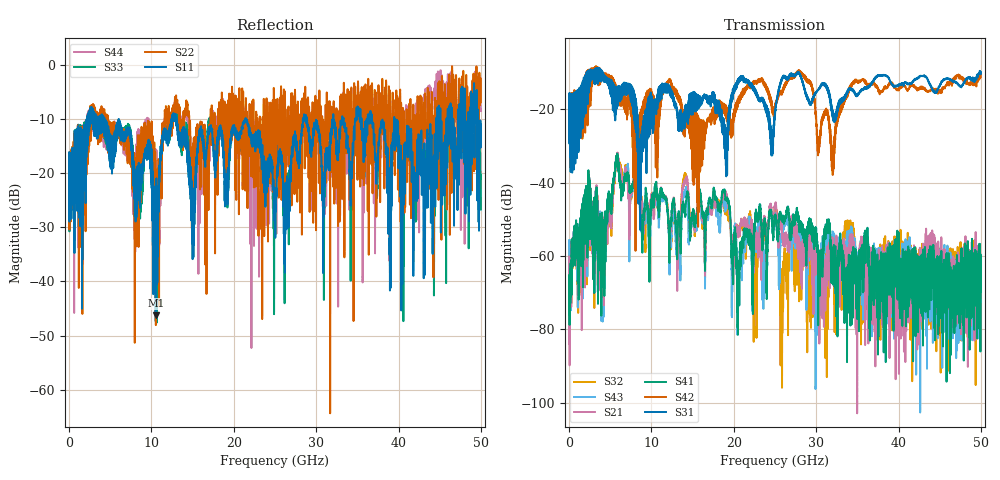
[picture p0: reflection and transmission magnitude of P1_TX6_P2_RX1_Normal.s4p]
!Keysight Technologies,N5225B,MY57041031,A.13.20.10
!Date: Friday, May 31, 2019 11:28:39
!Correction: S11(Full 4 Port(1,2,3,4))
!S12(Full 4 Port(1,2,3,4))
!S13(Full 4 Port(1,2,3,4))
!S14(Full 4 Port(1,2,3,4))
!S21(Full 4 Port(1,2,3,4))
!S22(Full 4 Port(1,2,3,4))
!S23(Full 4 Port(1,2,3,4))
!S24(Full 4 Port(1,2,3,4))
!S31(Full 4 Port(1,2,3,4))
!S32(Full 4 Port(1,2,3,4))
!S33(Full 4 Port(1,2,3,4))
!S34(Full 4 Port(1,2,3,4))
!S41(Full 4 Port(1,2,3,4))
!S42(Full 4 Port(1,2,3,4))
!S43(Full 4 Port(1,2,3,4))
!S44(Full 4 Port(1,2,3,4))
!S4P File: Measurements: <S11,S12,S13,S14>,
!<S21,S22,S23,S24>,
!<S31,S32,S33,S34>,
!<S41,S42,S43,S44>:
# Hz S  dB  R 50.0
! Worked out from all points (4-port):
!   5000 points, 10 MHz to 50 GHz, reference 50 ohm
!   strongest paths, dB at 10 MHz, 12.51 GHz, 25.01 GHz, 37.51 GHz, 50 GHz:
!     S31: -19.4, -15.4, -21.6, -10.8, -9.9
!     S42: -19.4, -14.2, -20.1, -14.4, -10.4
!     S41: -66.7, -46.4, -49.3, -86.8, -69.7
!     S21: -60.2, -47.1, -46.7, -66.3, -60.9
!     S43: -55.6, -50.4, -48.8, -64.3, -72.6
!     S32: -58.5, -49.6, -47.2, -77.7, -63.2
!   lowest |S11| = -46.2 dB at 10.52 GHz (marker M1), VSWR 1.01, Z = 49.5 - j0.0828 ohm
!   |S11| at or under -10 dB: 4.286 GHz to 12.47 GHz (8.179 GHz wide, 97.6 % of centre); 13.02 GHz to 21.43 GHz (8.402 GHz wide, 48.8 % of centre); 21.46 GHz to 28.39 GHz (6.925 GHz wide, 27.8 % of centre)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
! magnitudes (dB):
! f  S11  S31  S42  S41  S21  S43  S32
! 10 MHz  -19.4  -19.4  -19.4  -66.7  -60.2  -55.6  -58.5
! 5.85 GHz  -13.7  -19.2  -15.9  -32.1  -31.9  -32.3  -32.3
! 10.52 GHz  -46.2  -18.4  -22.4  -41.7  -42.7  -42.6  -44.0
! 12.81 GHz  -9.1  -17.9  -15.5  -46.7  -46.1  -51.0  -49.7
! 28.05 GHz  -15.2  -10.8  -9.7  -52.4  -57.1  -54.3  -63.7
! 32.01 GHz  -11.7  -21.2  -37.9  -63.3  -57.4  -53.3  -58.4
! 50 GHz  -11.0  -9.9  -10.4  -69.7  -60.9  -72.6  -63.2
